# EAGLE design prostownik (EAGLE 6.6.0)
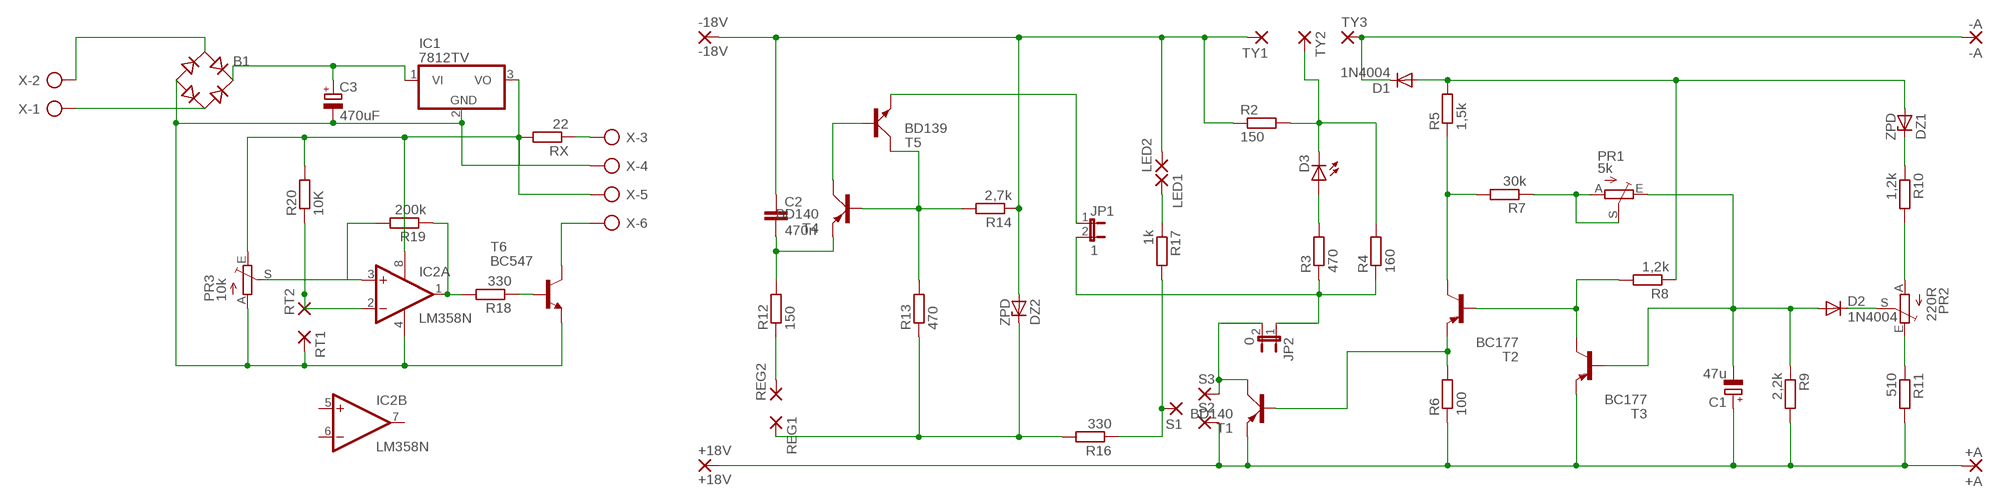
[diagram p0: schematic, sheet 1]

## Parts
+18V  +18V  2,54/0,8  [2,54/0,8]
+A  +A  2,54/0,8  [2,54/0,8]
-18V  -18V  2,54/0,8  [2,54/0,8]
-A  -A  2,54/0,8  [2,54/0,8]
B1  RB1A  [RB1A]
C1  47u  CPOL-EUE2-4  [E2-4]
C2  470n  C-EU050-025X075  [C050-025X075]
C3  470uF  CPOL-EUE5-13  [E5-13]
D1  1N4004  [DO41-10]
D2  1N4004  [DO41-10]
D3  LED5MM  [LED5MM]
DZ1  ZPD  [DO35Z10]
DZ2  ZPD  [DO35Z10]
IC1  7812TV  [TO220V]
IC2  LM358N  [DIL08]
JP1  1  JP1E  [JP1]
JP2  0  JP1E  [JP1]
LED1  2,15/1,0  [2,15/1,0]
LED2  2,15/1,0  [2,15/1,0]
PR1  5k  TRIM_EU-CA9V  [CA9V]
PR2  220R  TRIM_EU-CA9V  [CA9V]
PR3  10k  TRIM_EU-CA9V  [CA9V]
R2  150  R-EU_0207/10  [0207/10]
R3  470  R-EU_0207/10  [0207/10]
R4  160  R-EU_0207/10  [0207/10]
R5  1,5k  R-EU_0207/10  [0207/10]
R6  100  R-EU_0207/10  [0207/10]
R7  30k  R-EU_0207/10  [0207/10]
R8  1,2k  R-EU_0207/10  [0207/10]
R9  2,2k  R-EU_0207/10  [0207/10]
R10  1,2k  R-EU_0207/10  [0207/10]
R11  510  R-EU_0207/10  [0207/10]
R12  150  R-EU_0207/10  [0207/10]
R13  470  R-EU_0207/10  [0207/10]
R14  2,7k  R-EU_0207/10  [0207/10]
R16  330  R-EU_0207/10  [0207/10]
R17  1k  R-EU_0207/10  [0207/10]
R18  330  R-EU_0207/10  [0207/10]
R19  200k  R-EU_0207/10  [0207/10]
R20  10K  R-EU_0207/10  [0207/10]
REG1  2,15/1,0  [2,15/1,0]
REG2  2,15/1,0  [2,15/1,0]
RT1  2,15/1,0  [2,15/1,0]
RT2  2,15/1,0  [2,15/1,0]
RX  22  R-EU_0207/10  [0207/10]
S1  2,15/1,0  [2,15/1,0]
S2  2,15/1,0  [2,15/1,0]
S3  2,15/1,0  [2,15/1,0]
T1  BD140  [TO126AV]
T2  BC177  [TO18]
T3  BC177  [TO18]
T4  BD140  [TO126AV]
T5  BD139  [TO126AV]
T6  BC547  [TO92]
TY1  2,15/1,0  [2,15/1,0]
TY2  2,15/1,0  [2,15/1,0]
TY3  2,15/1,0  [2,15/1,0]
X  AK500/6-H  [AK500/6-H]

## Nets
+A: +18V.1(P) +A.1(P) C1.+ R6.1 R9.2 R11.2 S2.1(P) T1.E T3.1(E)
-18V: -18V.1(P) C2.1 DZ2.A LED2.1(P) R2.1 R14.1 TY1.1(P)
N$1: T4.C T5.B
N$2: C2.2 R12.2 T4.E
N$3: R12.1 REG2.1(P)
N$4: R13.2 R14.2 T4.B T5.C
N$5: R5.1 R7.2 T2.3(C)
N$6: PR1.A PR1.S R7.1
N$7: R16.1 R17.2 S1.1(P)
N$8: LED1.1(P) R17.1
N$9: JP1.1 T5.E
N$10: JP1.2 JP2.1 R3.1 R4.1
N$11: D3.A R3.2
N$12: JP2.2 S3.1(P) T1.C
N$13: PR2.E R11.1
N$14: PR2.A R10.2
N$15: DZ1.C R10.1
N$16: B1.AC1 X.2
N$17: D1.A DZ1.A R5.2 R8.1
N$18: B1.AC2 X.1
N$19: B1.+ C3.+ IC1.1(VI)
N$20: C1.- D2.A PR1.E R9.1 T3.2(B)
N$21: D2.C PR2.S
N$22: R8.2 T2.2(B) T3.3(C)
N$23: RX.1 X.3
N$24: R6.2 T1.B T2.1(E)
N$25: T6.3(C) X.6
N$26: IC1.3(VO) IC2.8(P:V+) PR3.E R20.2 RX.2 X.5
N$27: R18.1 T6.2(B)
N$28: IC2.1(A:OUT) R18.2 R19.1
N$29: IC2.3(A:+IN) PR3.S R19.2
N$30: B1.- C3.- IC1.2(GND) IC2.4(P:V-) PR3.A RT1.1(P) T6.1(E) X.4
N$31: IC2.2(A:-IN) R20.1 RT2.1(P)
REG1: DZ2.C R13.1 R16.2 REG1.1(P)
TY2: D3.K(C) R2.2 R4.2 TY2.1(P)
TY3: -A.1(P) D1.C TY3.1(P)
Unconnected: IC2.5(B:+IN) IC2.6(B:-IN) IC2.7(B:OUT)

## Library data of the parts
+18V +A -18V -A = wirepad:2,54/0,8: THROUGH-HOLE PAD
B1 = rectifier:RB1A: RECTIFIER 1 A
C1 = resistor:CPOL-EU: POLARIZED CAPACITOR, European symbol
C2 = resistor:C-EU: CAPACITOR, European symbol
C3 = rcl:CPOL-EU: POLARIZED CAPACITOR, European symbol
D1 D2 = diode:1N4004: DIODE
D3 = led:LED: LED
DZ1 DZ2 = diode:ZPD: Z DIODE
IC1 = linear:78*: Positive VOLTAGE REGULATOR Source: http://cache.national.com/ds/LM/LM78L05.pdf http://www.fairchildsemi.com/ds/LM/LM7805.pdf
IC2 = linear:LM358: OP AMP also LM158; LM258; LM2904 Source: http://cache.national.com/ds/LM/LM158.pdf
JP1 JP2 = jumper:JP1E: JUMPER
LED1 LED2 REG1 REG2 RT1 RT2 S1-S3 TY1-TY3 = wirepad:2,15/1,0: THROUGH-HOLE PAD
PR1-PR3 = pot:TRIM_EU-: POTENTIOMETER
R2-R14 R16-R20 RX = resistor:R-EU_: RESISTOR, European symbol
T1 T4 = transistor-power:BD140: PNP TRANSISTOR
T2 T3 = transistor-pnp:BC177*: PNP Transistor
T5 = transistor-power:BD139: NPN TRANSISTOR
T6 = transistor-neu-to92:BC547: NPN TRANSISTOR
X = con-ptr500:AK500/6-H: CONNECTOR Aug. 2004 / PTR Meßtechnik: Die Bezeichnung der Serie AK505 wurde geändert. Es handelt sich hierbei um AK500 in horizontaler Ausführung.

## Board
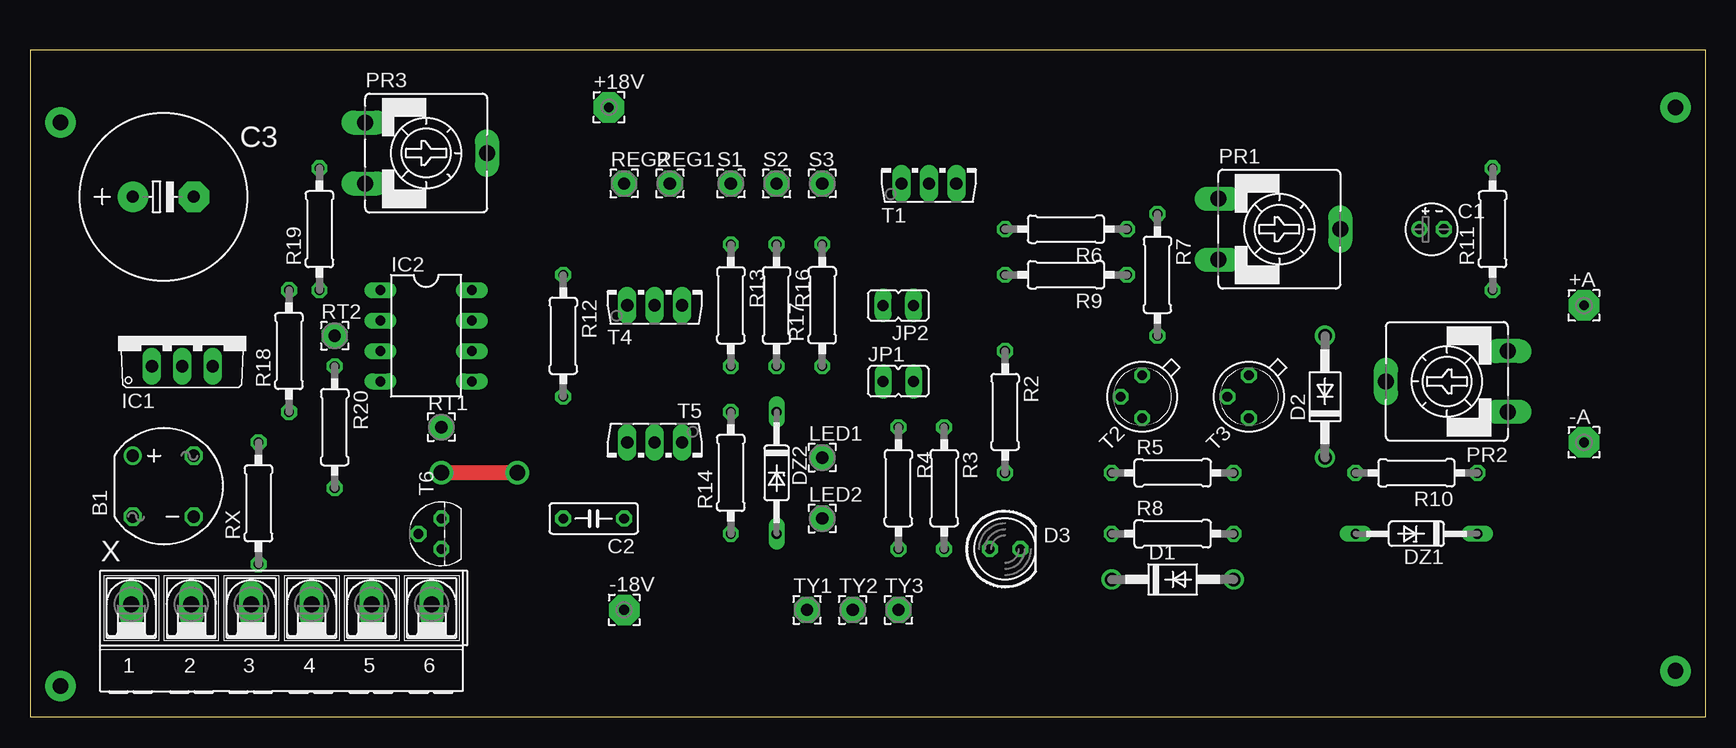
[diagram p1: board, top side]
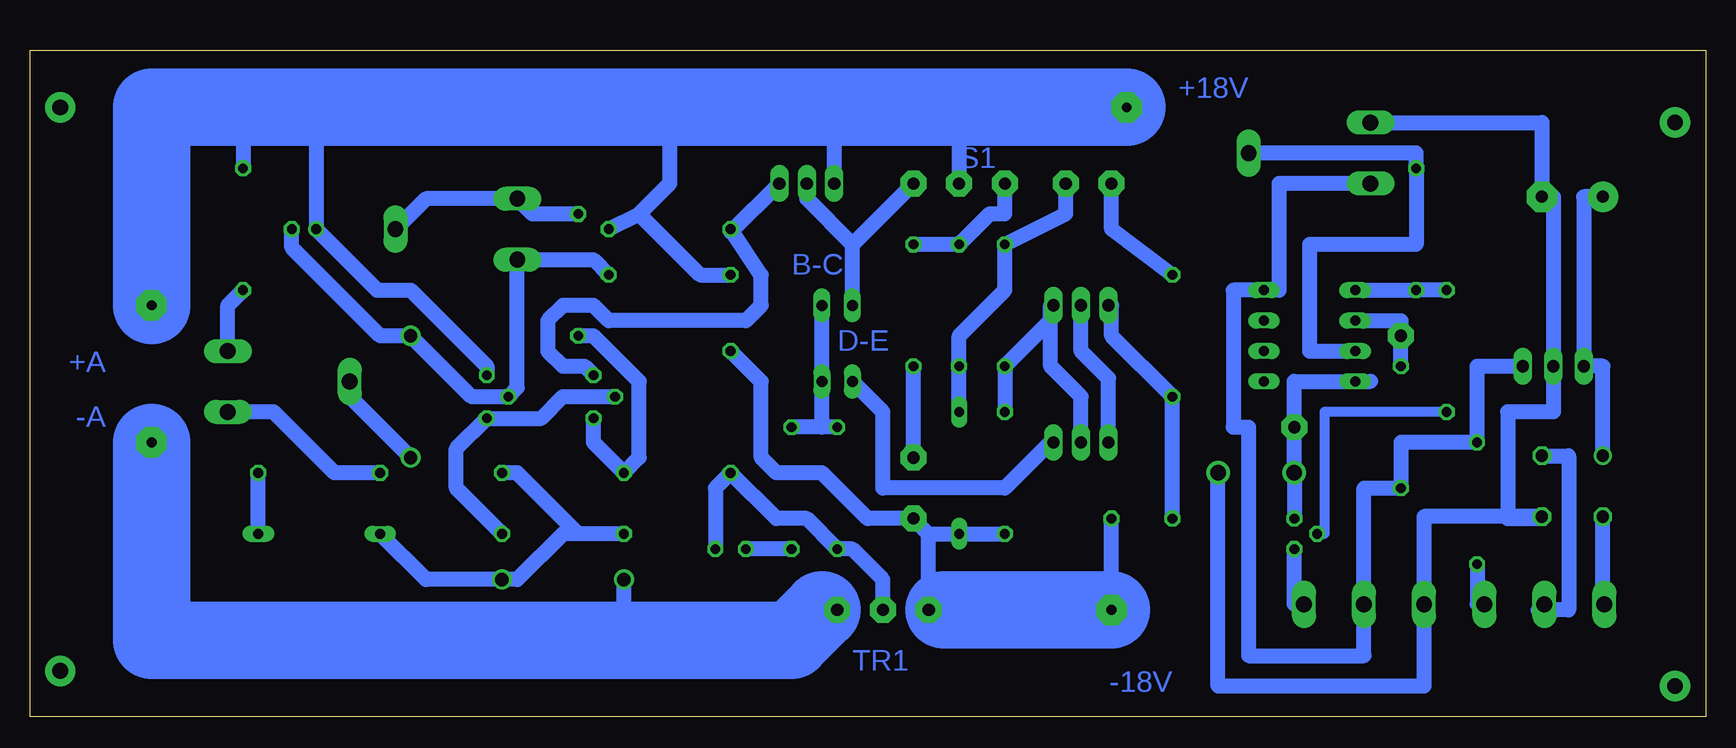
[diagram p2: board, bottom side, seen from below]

Size 139.68 x 55.55 mm. Coordinates in mm from the lower left corner, seen from the top.
Outline: 0,0 139.68,0 139.68,55.55 0,55.55 0,0
Copper layers (1*16): Top 0.035mm / dielectric 1.5mm / Bottom 0.035mm
Design rules "default": minimum track width 10mil, minimum drill 24mil, track to track 8mil, track to pad 8mil, pad to pad 8mil, via to via 8mil, smd to smd 8mil, copper to edge 40mil, drill to drill 8mil, minimum pad ring 10mil, minimum via ring 8mil, stop-mask expansion 4mil, vias tented up to drill 0mil, thermal gap 10mil

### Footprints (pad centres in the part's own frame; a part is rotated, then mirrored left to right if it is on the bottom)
2,54/0,8 = drill 0.813 pad 2.54 octagon: 1 0,0
RB1A = drill 1.016: + -2.54,2.54 | drill 1.016 octagon: - 2.54,-2.54; AC1 2.54,2.54; AC2 -2.54,-2.54
E2-4 = drill 0.813 pad 1.27: + -1.016,0 | drill 0.813 pad 1.27 octagon: - 1.016,0
C050-025X075 = drill 0.813 octagon: 1 -2.54,0; 2 2.54,0
E5-13 = drill 1.016 pad 2.54: + -2.54,0 | drill 1.016 pad 2.54 octagon: - 2.54,0
DO41-10 = drill 1.118: A 5.08,0; C -5.08,0
LED5MM = drill 0.813 octagon: A -1.27,0; K 1.27,0
DO35Z10 = drill 0.813 long: A 5.08,0; C -5.08,0
TO220V = drill 1.016 long: 1 -2.54,-2.54; 2 0,-2.54; 3 2.54,-2.54
DIL08 = drill 0.813 long: 1 -3.81,-3.81; 2 -1.27,-3.81; 3 1.27,-3.81; 4 3.81,-3.81; 5 3.81,3.81; 6 1.27,3.81; 7 -1.27,3.81; 8 -3.81,3.81
JP1 = drill 0.914 long: 1 0,-1.27; 2 0,1.27
2,15/1,0 = drill 1.016 pad 2.159 octagon: 1 0,0
CA9V = drill 1.321 long: A -2.54,-5.08; E 2.54,-5.08; S 0,5.08
0207/10 = drill 0.813 octagon: 1 -5.08,0; 2 5.08,0
TO126AV = drill 1.016 long: B 2.286,-1.27; C 0,-1.27; E -2.286,-1.27
TO18 = drill 0.813 octagon: 1 -1.27,-1.27; 2 1.27,-1.27; 3 1.27,1.27
TO92 = drill 0.813 octagon: 1 1.27,0; 2 0,1.905; 3 -1.27,0
AK500/6-H = drill 1.321 long: 1 -12.522,0; 2 -7.518,0; 3 -2.515,0; 4 2.515,0; 5 7.518,0; 6 12.522,0

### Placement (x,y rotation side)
+18V  48.26,50.8 0.1 top
+A  129.54,34.29 0 top
-18V  49.53,8.89 0 top
-A  129.54,22.86 0 top
B1  11.11,19.21 0 top
C1  116.84,40.64 0 top
C2  46.99,16.51 180 top
C3  11.11,43.35 0 top
D1  95.25,11.43 0 top
D2  107.95,26.67 90 top
D3  81.28,13.97 0 top
DZ1  115.57,15.24 180 top
DZ2  62.23,20.32 270 top
IC1  12.7,31.75 0 top
IC2  33.02,31.75 270 top
JP1  72.39,27.94 270 top
JP2  72.39,34.29 90 top
LED1  66.04,21.59 0 top
LED2  66.04,16.51 0 top
PR1  104.14,40.64 270 top
PR2  118.11,27.94 90 top
PR3  33.02,46.99 270 top
R2  81.28,25.4 270 top
R3  76.2,19.05 270 top
R4  72.39,19.05 270 top
R5  95.25,20.32 0 top
R6  86.36,40.64 180 top
R7  93.98,36.83 270 top
R8  95.25,15.24 0 top
R9  86.36,36.83 180 top
R10  115.57,20.32 180 top
R11  121.92,40.64 90 top
R12  44.45,31.75 270 top
R13  58.42,34.29 270 top
R14  58.42,20.32 90 top
R16  62.23,34.29 270 top
R17  66.04,34.29 90 top
R18  21.59,30.48 90 top
R19  24.13,40.64 90 top
R20  25.4,24.13 270 top
REG1  53.34,44.45 0 top
REG2  49.53,44.45 0 top
RT1  34.29,24.13 0 top
RT2  25.4,31.75 0 top
RX  19.05,17.78 90 top
S1  58.42,44.45 0 top
S2  62.23,44.45 0 top
S3  66.04,44.45 0 top
T1  74.93,45.72 0 top
T2  92.71,26.67 225 top
T3  101.6,26.67 225.2 top
T4  52.07,35.56 0 top
T5  52.07,21.59 180 top
T6  34.29,15.24 90 top
TY1  64.77,8.89 0 top
TY2  68.58,8.89 0 top
TY3  72.39,8.89 0 top
X  20.96,9.36 0 top

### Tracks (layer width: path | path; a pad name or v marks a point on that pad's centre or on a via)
+A
  Bottom 1.27: 62.23,50.8 S2.1 | T1.E 72.64,50.55 72.39,50.8 | 88.9,41.91 86.36,44.45 86.36,50.8 | 88.9,41.91 R6.1 | R9.2 83.82,36.83 88.9,41.91 | 121.92,50.8 R11.2 | 115.57,50.8 115.82,50.55 C1.+ 110.74,35.56 107.95,35.56 101.59,29.2 T3.1
  Bottom 6.452: +18V.1 62.23,50.8 72.39,50.8 86.36,50.8 115.57,50.8 121.92,50.8 129.54,50.8 +A.1
-18V
  Bottom 1.27: -18V.1 C2.1 | R14.1 DZ2.A 64.77,15.24 | 64.77,15.24 LED2.1 69.85,16.51 73.66,20.32 77.47,20.32 78.74,21.59 78.74,27.94 R2.1 | 64.77,15.24 TY1.1 63.5,8.89
  Bottom 6.452: -18V.1 63.5,8.89
N$1
  Bottom 1.27: T5.B 49.78,28.19 52.07,30.48 T4.C
N$2
  Bottom 1.27: C2.2 R12.2 49.53,31.75 49.53,34.29 T4.E
N$3
  Bottom 1.27: R12.1 49.53,40.64 REG2.1
N$4
  Bottom 0.254: 54.61,34.29 T4.B
  Bottom 1.27: R14.2 R13.2 54.61,33.02 | T5.C 52.07,26.67 54.61,29.21 54.61,33.02 | 54.61,33.02 54.61,34.29
N$5
  Bottom 1.27: T2.3 92.71,22.86 R5.1 88.9,21.59 88.9,27.94 92.71,31.75 R7.2
N$6
  Bottom 1.27: R7.1 97.79,41.91 PR1.A 106.68,43.18 PR1.S
N$7
  Bottom 1.27: S1.1 58.42,41.91 59.69,41.91 R16.1 R17.2
N$8
  Bottom 1.27: LED1.1 R17.1
N$9
  Bottom 1.27: T5.E 54.61,22.86 58.42,19.05 68.58,19.05 68.58,25.4 JP1.1
N$10
  Bottom 1.27: JP2.1 JP1.2 73.66,24.13 | R4.1 73.66,24.13 | 73.66,24.13 R3.1
N$11
  Bottom 1.27: R3.2 D3.A
N$12
  Bottom 1.27: 71.12,39.37 S3.1 | JP2.2 71.12,39.37 | T1.C 74.93,43.18 71.12,39.37
N$13
  Bottom 1.27: PR2.E 123.19,34.29 R11.1
N$14
  Bottom 1.27: R10.2 114.3,20.32 119.38,25.4 PR2.A
N$15
  Bottom 1.27: DZ1.C R10.1
N$16
  Bottom 1.27: B1.AC1 11.43,21.75 11.43,8.89 13.44,8.89 | 13.97,8.89 13.44,8.89 | 13.44,8.89 X.2
N$17
  Bottom 1.27: DZ1.A 106.68,11.43 D1.A 99.06,11.43 95.25,15.24 93.98,15.24 | R8.1 93.98,15.24 | R5.2 99.06,20.32 93.98,15.24
N$18
  Bottom 1.27: X.1 8.57,9.36 B1.AC2
N$19
  Bottom 1.27: B1.+ 8.57,29.21 IC1.1 10.16,43.35 C3.+
N$20
  Bottom 1.27: C1.- 117.86,39.12 110.49,31.75 D2.A 102.86,26.66 T3.2 99.06,27.41 PR1.E 92.71,38.1 R9.1
N$21
  Bottom 1.27: PR2.S 113.03,26.67 D2.C
N$22
  Bottom 1.27: R8.2 104.14,19.05 104.14,22.34 T3.3 97.05,24.87 95.25,26.67 T2.2
N$23
  Bottom 1.27: RX.1 19.05,9.36 X.3
N$24
  Bottom 1.27: T1.B 81.28,40.39 R6.2 78.74,36.83 78.74,34.29 80.01,33.02 91.44,33.02 92.71,34.29 95.25,34.29 96.52,33.02 96.52,30.48 95.25,29.21 93.45,29.21 T2.1
N$25
  Bottom 1.27: X.6 34.29,9.36 T6.3
N$26
  Bottom 1.27: IC1.3 19.05,29.21 RX.2 25.4,22.86 R20.2 28.48,19.05 X.5 28.48,5.08 38.1,5.08 38.1,24.13 39.37,24.13 39.37,35.56 IC2.8 35.56,35.56 35.56,44.45 PR3.E
N$27
  Bottom 0.813: T6.2 31.75,15.24 31.75,25.4 R18.1
N$28
  Bottom 1.27: R18.2 R19.1 IC2.1
N$29
  Bottom 1.27: PR3.S 24.13,46.99 R19.2 24.13,39.37 33.02,39.37 33.02,30.48 IC2.3
N$30  (via drill 1.3 pad 0.25)
  Top 1.27: v40.64,20.32 v34.29,20.32
  Bottom 1.27: PR3.A 13.65,49.53 C3.- 12.7,43.35 IC1.2 12.7,25.4 16.51,25.4 16.51,16.51 13.65,16.51 B1.- 23.48,16.67 X.4 23.48,2.54 40.64,2.54 v40.64,20.32 | 27.94,27.94 IC2.4 34.29,27.94 RT1.1 v34.29,20.32 T6.1
N$31
  Bottom 1.27: IC2.2 25.4,33.02 RT2.1 R20.1
N$32  (via drill 1.3 pad 2.54)
  other vias: 2.54,49.53
N$33  (via drill 1.3 pad 2.54)
  other vias: 2.54,2.54
N$34  (via drill 1.3 pad 2.54)
  other vias: 137.16,3.81
N$35  (via drill 1.3 pad 2.54)
  other vias: 137.16,50.8
REG1
  Bottom 1.27: REG1.1 53.34,41.91 R13.1 58.42,35.56 62.23,31.75 R16.2 DZ2.C
TY2
  Bottom 1.27: D3.K 82.55,19.05 R2.2 77.47,16.51 74.93,16.51 R4.2 71.12,13.97 68.58,11.43 TY2.1
TY3
  Bottom 0.254: TY3.1 73.66,8.89
  Bottom 1.27: 90.17,6.35 D1.C
  Bottom 6.452: -A.1 129.54,6.35 90.17,6.35 76.2,6.35 73.66,8.89

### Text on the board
Bottom: +18V | S1 | B-C | D-E | +A | -A | -18V | TR1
